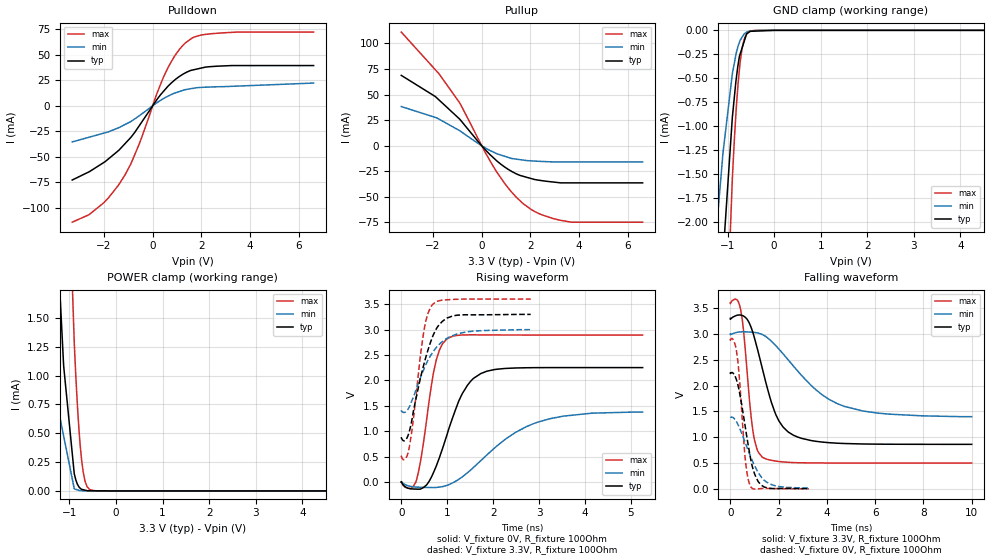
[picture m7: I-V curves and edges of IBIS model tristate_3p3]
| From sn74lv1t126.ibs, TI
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|   tristate_3p3 Model
[Model]   tristate_3p3
Model_type   3-state
Polarity   Non-Inverting
Vmeas = 1.65
Vref = 0
Cref = 30pF
Rref = 150
|   typ   min   max
|   (nom PVT)   (fast PVT)   (slow PVT)
C_comp   2.364e-12   2.330e-12   2.404e-12
| Where nom  PVT is Nominal Process, 3.3V, 40C
|   Fast PVT is Strong Process,  3.6V, -40C
|   Slow PVT is Weak Process,   3V, 140C
[Voltage Range]   3.3   3   3.6
|Junction Temperature
[Temperature Range]   40   140   -40
[Pullup Reference]   3.3   3   3.6
[Pulldown Reference]   0   0   0
[Power Clamp Reference]   3.3   3   3.6
[GND Clamp Reference]   0   0   0
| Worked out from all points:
|   slope of the pulldown table from 0 to 0.495 V, typ, clamps not added: 31.9 ohm
|   slope of the pullup table from 0 to 0.495 V, typ, clamps not added: 41 ohm
|   GND clamp passes 1 mA (typ) near -0.91 V on its own axis
|   POWER clamp passes 1 mA (typ) near -1.10 V on its own axis
|   falling waveform, V_fixture 3.3V, R_fixture 100Ohm: 20-80 % time 914ps typ, 2.08ns min, 372ps max; typ from 3.3 V to 0.861 V
|   rising waveform, V_fixture 0V, R_fixture 100Ohm: 20-80 % time 552ps typ, 1.19ns min, 290ps max; typ from 0 V to 2.25 V
|   rising waveform, V_fixture 3.3V, R_fixture 100Ohm: 20-80 % time 406ps typ, 512ps min, 248ps max; typ from 0.861 V to 3.3 V
|   falling waveform, V_fixture 0V, R_fixture 100Ohm: 20-80 % time 494ps typ, 750ps min, 274ps max; typ from 2.25 V to 0.004 V
[Pulldown]
|   Voltage   I(typ)   I(min)   I(max)
-3.3V     -72.82mA   -35.47mA   -114.2mA
-2.617V   -64.87mA   -30.92mA   -106.9mA
-2.009V   -55.7mA    -26.87mA   -95.21mA
-1.138V   -37.26mA   -18.43mA   -67.92mA
-536.4mV  -19.09mA   -9.58mA    -36.57mA
172.8mV   6.039mA    2.968mA    11.96mA
478.8mV   15.08mA    7.505mA    29.95mA
882mV     24.79mA    12.24mA    48.03mA
1.336V    32.19mA    15.79mA    61.53mA
1.706V    35.42mA    17.31mA    67.42mA
2.473V    38.52mA    18.5mA     70.78mA
6.6V      39.41mA    22.25mA    72.23mA
[GND Clamp]
|   Voltage   I(typ)   I(min)   I(max)
-3.3V     -38.99mA   -22.04mA   -61.06mA
-1.32V    -4.448mA   -2.546mA   -7.881mA
-1.132V   -2.608mA   -1.471mA   -4.674mA
-1.098V   -2.363mA   -1.278mA   -4.096mA
-897.6mV  -910.4uA   -455.1uA   -1.553mA
-818.4mV  -523.8uA   -248.8uA   -854.5uA
-774mV    -359.6uA   -165uA     -555.8uA
-727.2mV  -243.1uA   -102.5uA   -323.5uA
-651.6mV  -128.5uA   -43.09uA   -107.2uA
-591mV    -36.58uA   -19.39uA   -39.82uA
-324mV    -6.368uA   -497.7nA   -128.7nA
6.6V      0A         0A         0A
[Pullup]
|   Voltage   I(typ)   I(min)   I(max)
-3.3V     68.77mA    38.29mA    111.1mA
-1.904V   48.1mA     27.67mA    74.31mA
-1.757V   44.85mA    26.05mA    70.44mA
-896.4mV  25.83mA    14.62mA    41.65mA
0V        0A         0A         0A
536.4mV   -12.99mA   -6.868mA   -22.63mA
1.091V    -23.16mA   -11.42mA   -41.42mA
1.706V    -29.9mA    -14.03mA   -56.68mA
2.012V    -31.96mA   -14.75mA   -62.04mA
2.473V    -34.13mA   -15.35mA   -67.58mA
3.683V    -36.28mA   -15.84mA   -74.71mA
6.6V      -36.28mA   -15.84mA   -74.71mA
[POWER Clamp]
|   Voltage   I(typ)   I(min)   I(max)
-3.3V     36.75mA    19.76mA    64.19mA
-1.634V   5.953mA    2.712mA    13.77mA
-1.383V   3.146mA    1.163mA    8.47mA
-1.323V   2.664mA    875.7uA    7.391mA
-1.12V    1.063mA    466.1uA    3.951mA
-897mV    149.2uA    17.77uA    1.284mA
-820.8mV  51.68uA    7.853uA    684.8uA
-781.2mV  27.96uA    3.662uA    452.8uA
-745.2mV  14.7uA     2.193uA    290.8uA
-666mV    6.558uA    668nA      84.87uA
-561.6mV  1.392uA    199.1nA    10.67uA
6.6V      0A         0A         0A
[Ramp]
R_load = 100
|   typ   min   max
dV/dt_r   1.35145/5.4848e-10   0.837092/1.2267e-09   1.73601/2.87803e-10
dV/dt_f   1.46338/9.10671e-10   0.961975/2.07762e-09   1.86042/3.70621e-10
[Falling Waveform]
V_fixture = 3.3V
V_fixture_min = 3V
V_fixture_max = 3.6V
R_fixture = 100Ohm
|   Time   V(typ)   V(min)   V(max)
0s        3.3V       3V         3.6V
254ps     3.357V     3.028V     3.668V
422ps     3.365V     3.04V      3.484V
548ps     3.346V     3.041V     3.067V
934ps     3.029V     3.032V     1.128V
1.33ns    2.324V     2.987V     610.5mV
2.01ns    1.317V     2.708V     529.2mV
2.788ns   1.003V     2.282V     505.6mV
4.724ns   877.1mV    1.596V     499.4mV
9.998ns   861mV      1.397V     499.3mV
[Rising Waveform]
V_fixture = 0V
V_fixture_min = 0V
V_fixture_max = 0V
R_fixture = 100Ohm
|   Time   V(typ)   V(min)   V(max)
0s        715pV      11.39nV    969.9pV
192ps     -131.7mV   -85.03mV   -126.4mV
332ps     -139.7mV   -100.6mV   42.58mV
700ps     182.6mV    -109.6mV   2.146V
828ps     474.2mV    -100.2mV   2.592V
990ps     914.9mV    -66.9mV    2.815V
1.438ns   1.901V     179.7mV    2.897V
1.86ns    2.181V     530.2mV    2.896V
3.23ns    2.253V     1.245V     2.893V
5.254ns   2.253V     1.376V     2.893V
[Rising Waveform]
V_fixture = 3.3V
V_fixture_min = 3V
V_fixture_max = 3.6V
R_fixture = 100Ohm
|   Time   V(typ)   V(min)   V(max)
0s        861mV      1.391V     499.3mV
84ps      817.1mV    1.375V     452.5mV
166ps     966.6mV    1.463V     646.5mV
266ps     1.404V     1.679V     1.256V
492ps     2.315V     2.221V     2.966V
572ps     2.571V     2.382V     3.294V
684ps     2.867V     2.552V     3.498V
894ps     3.162V     2.763V     3.58V
1.128ns   3.272V     2.885V     3.594V
2.818ns   3.3V       3V         3.6V
[Falling Waveform]
V_fixture = 0V
V_fixture_min = 0V
V_fixture_max = 0V
R_fixture = 100Ohm
|   Time   V(typ)   V(min)   V(max)
0s        2.252V     1.376V     2.893V
154ps     2.217V     1.365V     2.853V
280ps     2.075V     1.279V     2.589V
374ps     1.884V     1.185V     2.156V
636ps     1.152V     871.4mV    501.6mV
722ps     900.8mV    763.9mV    227.4mV
830ps     612.8mV    637.4mV    56.53mV
1.058ns   230.1mV    399.6mV    -3.221mV
1.39ns    37.82mV    171.6mV    7.727mV
3.254ns   3.84mV     12.42mV    227.9uV
